TYPE UDT 1
AUTHOR : RAmann
FAMILY : KP
NAME : KPID
VERSION : 1.0


  STRUCT
   B_FC : BYTE ;	//familiy code
   B_ID1 : BYTE ;	//ID byte 1
   B_ID2 : BYTE ;	//ID byte 2
   B_ID3 : BYTE ;	//ID byte 3
   B_ID4 : BYTE ;	//ID byte 4
   B_ID5 : BYTE ;	//ID byte 5
   B_ID6 : BYTE ;	//ID byte 6
   B_CRC : BYTE ;	//CRC byte
  END_STRUCT ;
END_TYPE

DATA_BLOCK DB 1
TITLE =
AUTHOR : RAmann
FAMILY : KP
NAME : KPLIST
VERSION : 1.0


  STRUCT
   AUDT_KeyList : ARRAY  [1 .. 4 ] OF //list of known keys (insert your data here)
   UDT 1;
  END_STRUCT ;
BEGIN
   AUDT_KeyList[1].B_FC := B#16#1;
   AUDT_KeyList[1].B_ID1 := B#16#D5;
   AUDT_KeyList[1].B_ID2 := B#16#2F;
   AUDT_KeyList[1].B_ID3 := B#16#BF;
   AUDT_KeyList[1].B_ID4 := B#16#C;
   AUDT_KeyList[1].B_ID5 := B#16#0;
   AUDT_KeyList[1].B_ID6 := B#16#0;
   AUDT_KeyList[1].B_CRC := B#16#35;
   AUDT_KeyList[2].B_FC := B#16#0;
   AUDT_KeyList[2].B_ID1 := B#16#0;
   AUDT_KeyList[2].B_ID2 := B#16#0;
   AUDT_KeyList[2].B_ID3 := B#16#0;
   AUDT_KeyList[2].B_ID4 := B#16#0;
   AUDT_KeyList[2].B_ID5 := B#16#0;
   AUDT_KeyList[2].B_ID6 := B#16#0;
   AUDT_KeyList[2].B_CRC := B#16#0;
   AUDT_KeyList[3].B_FC := B#16#0;
   AUDT_KeyList[3].B_ID1 := B#16#0;
   AUDT_KeyList[3].B_ID2 := B#16#0;
   AUDT_KeyList[3].B_ID3 := B#16#0;
   AUDT_KeyList[3].B_ID4 := B#16#0;
   AUDT_KeyList[3].B_ID5 := B#16#0;
   AUDT_KeyList[3].B_ID6 := B#16#0;
   AUDT_KeyList[3].B_CRC := B#16#0;
   AUDT_KeyList[4].B_FC := B#16#0;
   AUDT_KeyList[4].B_ID1 := B#16#0;
   AUDT_KeyList[4].B_ID2 := B#16#0;
   AUDT_KeyList[4].B_ID3 := B#16#0;
   AUDT_KeyList[4].B_ID4 := B#16#0;
   AUDT_KeyList[4].B_ID5 := B#16#0;
   AUDT_KeyList[4].B_ID6 := B#16#0;
   AUDT_KeyList[4].B_CRC := B#16#0;
END_DATA_BLOCK

FUNCTION FC 1 : VOID
TITLE =Read Key-ID and find matching database entry
//IANYr_KeyList
//-------------
//This pointer must refer to a list of key-IDs. Since key-IDs have a size of 8
//bytes, the length of the addressed area must be a multiple of 8.
AUTHOR : RAmann
FAMILY : KP
NAME : KPCHECK
VERSION : 1.0


VAR_INPUT
  IANYr_KeyList : ANY ;	//pointer on table with known keys and user data [length N*UDT1; read]
  II_StartAddressIn : INT ;	//input start address of KeyPilot (according to HW-Config)
END_VAR
VAR_OUTPUT
  OI_EntryNumber : INT ;	//number of first matching entry in the table of known keys [0=no matching entry]
  O_KeyIsPresent : BOOL ;	//key is corretly applied to reading head [0=no key/1=key applied]
  O_KeyIsKnown : BOOL ;	//key is listed in the table of known keys [0=key not found/1=key found]
END_VAR
VAR_TEMP
  LADW_KeyID : ARRAY  [1 .. 2 ] OF //buffer for key-id
  DWORD ;
  LDW_AR1 : DWORD ;	//buffer for address register 1
  LI_RetVal : INT ;	//state information of SFC14 "DPRD_DAT"
  LI_DataNumber : INT ;	//numer of keys in table
  LI_LoopCounter : INT ;	//loop counter
  LW_Address : WORD ;	//input start address from HW-Config
  LW_DB : WORD ;	//number of DB with key table
END_VAR
BEGIN
NETWORK
TITLE =backup of address register

      TAR1  #LDW_AR1;

NETWORK
TITLE =clear out values

      CLR   ;
      =     #O_KeyIsPresent;
      =     #O_KeyIsKnown;

      L     0;
      T     #OI_EntryNumber;

NETWORK
TITLE =read key id

      L     #II_StartAddressIn; // type cast from INT to WORD
      T     #LW_Address;

      CALL SFC   14 (// read data from KeyPilot
           LADDR                    := #LW_Address,
           RET_VAL                  := #LI_RetVal,
           RECORD                   := #LADW_KeyID);

NETWORK
TITLE =key applied?

      O(    ;
      L     #LADW_KeyID[1];
      L     0;
      <>D   ;
      )     ;
      O(    ;
      L     #LADW_KeyID[2];
      L     0;
      <>D   ;
      )     ;
      =     #O_KeyIsPresent;
      SPBN  mend; // jump if no key is applied to reading head

NETWORK
TITLE =check pointer to data table

// get address of pointer
      L     P##IANYr_KeyList;
      LAR1  ;

// check data type
      L     B [AR1,P#1.0]; // data type stored in ANY-pointer
      L     2;
      <>I   ;
      SPB   mend; // jump if data type is not BYTE

// check length of data area
      L     W [AR1,P#2.0]; // repeat counter (area length) stored in ANY-pointer
      L     8; // size of key-id
      /I    ;
      T     #LI_DataNumber; // store integral result of division
      SRD   16; // move remainder to the right
      L     0;
      <>I   ;
      SPB   mend; // jump if length of data area is not a multiple of key-id size

// open DB
      L     0;
      L     W [AR1,P#4.0]; // number of DB stored in ANY-pointer
      ==I   ;
      SPB   mdb1; // jump if data area is not part of a DB
      T     #LW_DB;
      AUF   DB [#LW_DB];

// get address of data area
mdb1: L     D [AR1,P#6.0]; // Adresse im ANY-Zeiger
      LAR1  ;

NETWORK
TITLE =search loop

      L     #LI_DataNumber;
mnxt: T     #LI_LoopCounter;

      U(    ;
      L     #LADW_KeyID[1];
      L     D [AR1,P#0.0]; // key-id from data area, part 1
      ==D   ;
      )     ;
      U(    ;
      L     #LADW_KeyID[2];
      L     D [AR1,P#4.0]; // key-id from data area, part 2
      ==D   ;
      )     ;
      SPB   mok;

      L     64; // size of one key-id (8) moved 3 bits to the left for addressing (8<<3)
      +AR1  ; // get address of next key-id in data area

      L     #LI_LoopCounter;
      LOOP  mnxt;
      SPA   mend;

mok:  SET   ;
      =     #O_KeyIsKnown;

      L     #LI_DataNumber;
      L     #LI_LoopCounter;
      -I    ;
      L     1;
      +I    ;
      T     #OI_EntryNumber;

NETWORK
TITLE =restore address register

mend: LAR1  #LDW_AR1;

END_FUNCTION

ORGANIZATION_BLOCK OB 1
TITLE = "Main Program Sweep (Cycle)"
//2. ID-Checking
//--------------
//
//In this example the actual key at the KeyPilot is searched in a database of
//known keys. If the key matches with a database entry, the KeyPilot-LED will be
//set to green, otherwise to red.
//
//For testing you have to adapt the database (DB1, array AUDT_KeyList) by
//inserting the key-IDs you want to search for (e.g. in data view).
AUTHOR : RAmann
FAMILY : KP
NAME : KPMAIN
VERSION : 1.0


VAR_TEMP
  OB1_EV_CLASS : BYTE ;	//Bits 0-3 = 1 (Coming event), Bits 4-7 = 1 (Event class 1)
  OB1_SCAN_1 : BYTE ;	//1 (Cold restart scan 1 of OB 1), 3 (Scan 2-n of OB 1)
  OB1_PRIORITY : BYTE ;	//Priority of OB Execution
  OB1_OB_NUMBR : BYTE ;	//1 (Organization block 1, OB1)
  OB1_RESERVED_1 : BYTE ;	//Reserved for system
  OB1_RESERVED_2 : BYTE ;	//Reserved for system
  OB1_PREV_CYCLE : INT ;	//Cycle time of previous OB1 scan (milliseconds)
  OB1_MIN_CYCLE : INT ;	//Minimum cycle time of OB1 (milliseconds)
  OB1_MAX_CYCLE : INT ;	//Maximum cycle time of OB1 (milliseconds)
  OB1_DATE_TIME : DATE_AND_TIME ;	//Date and time OB1 started
END_VAR
BEGIN
NETWORK
TITLE =read key-ID and check database
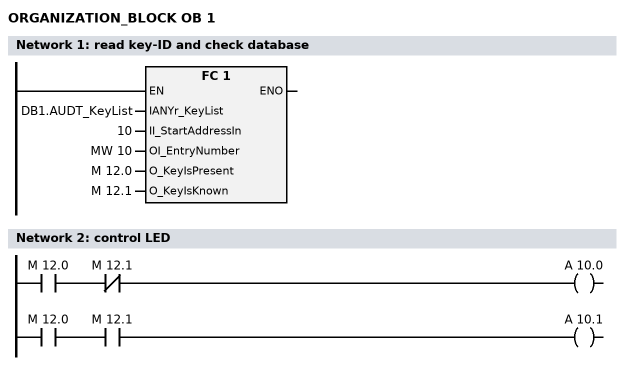
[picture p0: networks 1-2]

      CALL FC     1 (
           IANYr_KeyList            := DB1.AUDT_KeyList,
           II_StartAddressIn        := 10,
           OI_EntryNumber           := MW    10,
           O_KeyIsPresent           := M     12.0,
           O_KeyIsKnown             := M     12.1);

NETWORK
TITLE =control LED

// LED red: key present but unknown
      U     M     12.0;
      UN    M     12.1;
      =     A     10.0;

// LED green: key present and known
      U     M     12.0;
      U     M     12.1;
      =     A     10.1;

END_ORGANIZATION_BLOCK

